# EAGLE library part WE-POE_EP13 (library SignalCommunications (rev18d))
Power over Ethernet Transformer Characteristics Flyback transformer designed for PoE PDs Input voltage: 36 V to 57 V Switching frequencies: 200–500 kHz Operating temperature: –40 ºC to +125 ºC Insulation test voltage: 1.5 kVAC/1 min Different output powers and voltages available Applications Suitable for PoE IC’s like LTC4267, TPS 23750, TPS 23770, LM5070, LM 5071, LM 5072 Details see: http://katalog.we-online.de/en/pbs/WE-PoE? Updated by Dan Xu 2014-07-08 2014 (C) Wurth Elektronik
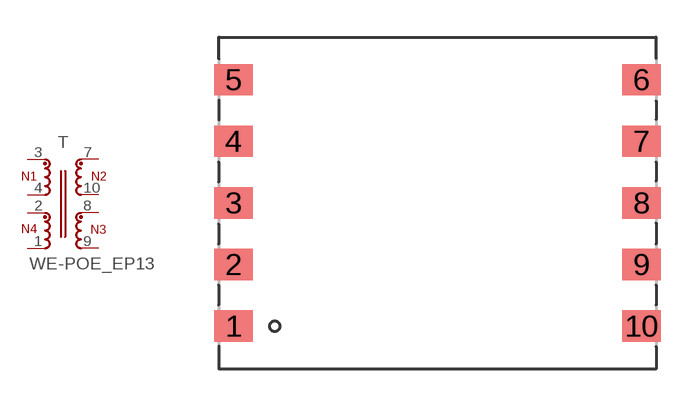
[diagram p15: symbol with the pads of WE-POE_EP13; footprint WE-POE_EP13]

Designator prefix T

## WE-POE_EP13_7491199112, WE-POE_EP13_7491199212, WE-POE_EP13_749119933, WE-POE_EP13_7491199331, WE-POE_EP13_749119950, WE-POE_EP13_7491199501  [WE-POE_EP13]
1  6  pas
2  7  pas
3  1  pas
4  8  pas
7  2  pas
8  4  pas
9  5  pas
10  3  pas

## Footprint WE-POE_EP13 (pad centres in mm)
smd 1.55 x 1.27: 1 -8.275,-5; 2 -8.275,-2.5; 3 -8.275,0; 4 -8.275,2.5; 5 -8.275,5; 6 8.275,5; 7 8.275,2.5; 8 8.275,0; 9 8.275,-2.5; 10 8.275,-5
